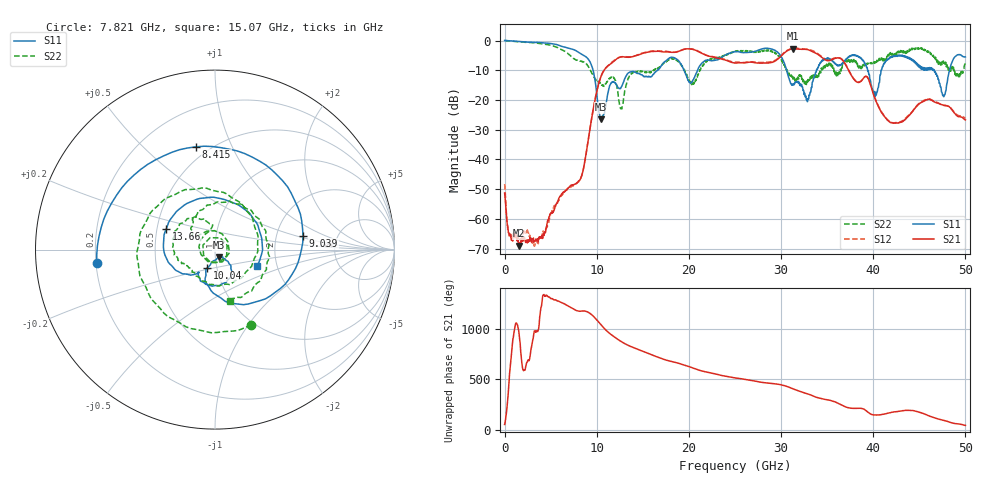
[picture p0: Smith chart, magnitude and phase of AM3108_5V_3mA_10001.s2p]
# Hz S DB R 50.0
!freq dBS11 angS11 dBS21 angS21 dBS12 angS12 dBS22 angS22
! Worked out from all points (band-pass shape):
!   1601 points, 10 MHz to 50 GHz, reference 50 ohm
!   highest |S21| = -2.77 dB at 31.28 GHz (marker M1); lowest = -69.0 dB at 1.603 GHz (marker M2)
!   |S21| within 3 dB of the highest: 12.37 GHz to 22.84 GHz (10.47 GHz wide, 59.5 % of centre); 29.81 GHz to 34.46 GHz (4.646 GHz wide, 14.5 % of centre)
!   lowest |S11| = -26.6 dB at 10.48 GHz (marker M3), VSWR 1.10, Z = 52 - j4.37 ohm
!   |S11| at or under -10 dB: 9.603 GHz to 16.59 GHz (6.991 GHz wide, 53.4 % of centre); 30.62 GHz to 33.84 GHz (3.228 GHz wide, 10 % of centre); 46.63 GHz to 48.28 GHz (1.655 GHz wide, 3.49 % of centre)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
!   |S22| runs from -23.0 to 0.0 dB; largest |S21 - S12| = 0.028
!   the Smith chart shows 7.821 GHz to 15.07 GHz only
!   S11 on the Smith chart (normalised r, x): 7.821 GHz: 0.20, -0.06; 8.415 GHz: 0.43, +0.74; 9.039 GHz: 2.84, +0.58; 10.04 GHz: 0.90, -0.19; 13.66 GHz: 0.56, +0.14; 15.07 GHz: 1.57, -0.30
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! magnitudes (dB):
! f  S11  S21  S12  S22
! 10 MHz  0.0  -51.3  -48.3  0.0
! 541.1 MHz  -0.1  -65.0  -65.4  -0.2
! 1.603 GHz  -0.4  -69.0  -66.7  -0.5
! 7.821 GHz  -3.6  -48.0  -48.0  -6.7
! 8.352 GHz  -4.6  -45.7  -45.7  -7.0
! 8.415 GHz  -4.7  -45.0  -45.1  -7.2
! 9.039 GHz  -6.1  -34.4  -34.3  -8.5
! 10.04 GHz  -19.0  -16.7  -16.7  -13.5
! 10.48 GHz  -26.6  -12.0  -12.0  -14.4
! 12.66 GHz  -15.7  -5.5  -5.5  -22.9
! 13.66 GHz  -10.6  -5.6  -5.5  -11.5
! 15.07 GHz  -12.1  -4.2  -4.1  -10.6
! 16.69 GHz  -9.7  -3.6  -3.5  -9.4
! 25 GHz  -3.8  -7.6  -7.3  -3.8
! 29.38 GHz  -3.4  -6.9  -6.6  -4.2
! 31.28 GHz  -15.0  -2.8  -2.7  -13.0
! 33.35 GHz  -15.6  -3.6  -3.3  -12.7
! 38 GHz  -4.8  -13.4  -13.3  -6.5
! 40.22 GHz  -18.8  -19.8  -19.5  -7.6
! 41.69 GHz  -6.1  -27.1  -27.0  -5.2
! 47.66 GHz  -18.9  -21.8  -21.8  -7.7
! 50 GHz  -5.5  -26.7  -26.2  -6.9
